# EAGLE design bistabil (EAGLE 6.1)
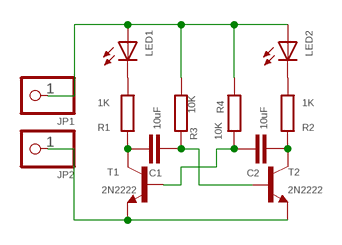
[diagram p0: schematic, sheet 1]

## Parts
C1  10uF  C-EU025-030X050  [C025-030X050]
C2  10uF  C-EU025-030X050  [C025-030X050]
JP1  PINHD-1X1  [1X01]
JP2  PINHD-1X1  [1X01]
LED1  LED3MM  [LED3MM]
LED2  LED3MM  [LED3MM]
R1  1K  R-EU_0204/7  [0204/7]
R2  1K  R-EU_0204/7  [0204/7]
R3  10K  R-EU_0204/7  [0204/7]
R4  10K  R-EU_0204/7  [0204/7]
T1  2N2222  [TO92-EBC-OVAL]
T2  2N2222  [TO92-EBC-OVAL]

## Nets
GND: JP2.1 T1.E T2.E
N$1: C1.1 R1.1 T1.C
N$2: LED1.K(C) R1.2
N$3: C2.2 R2.1 T2.C
N$5: C2.1 R4.1 T1.B
N$6: LED2.K(C) R2.2
N$8: JP1.1 LED1.A LED2.A R3.2 R4.2
N$12: C1.2 R3.1 T2.B

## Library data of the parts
C1 C2 = rcl:C-EU: CAPACITOR, European symbol
JP1 JP2 = pinhead:PINHD-1X1: PIN HEADER
LED1 LED2 = adafruit:LED: LED
R1-R4 = resistor:R-EU_: RESISTOR, European symbol
T1 T2 = adafruit:2N2222: NPN TRANSISTOR Big oval pads

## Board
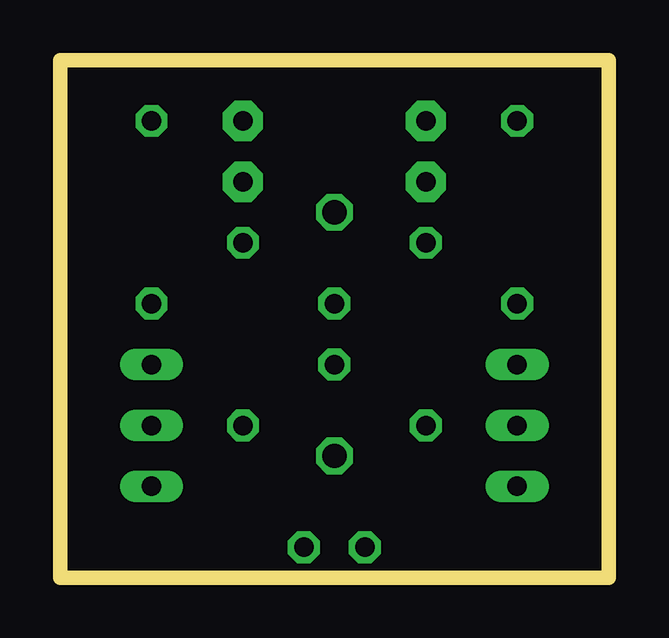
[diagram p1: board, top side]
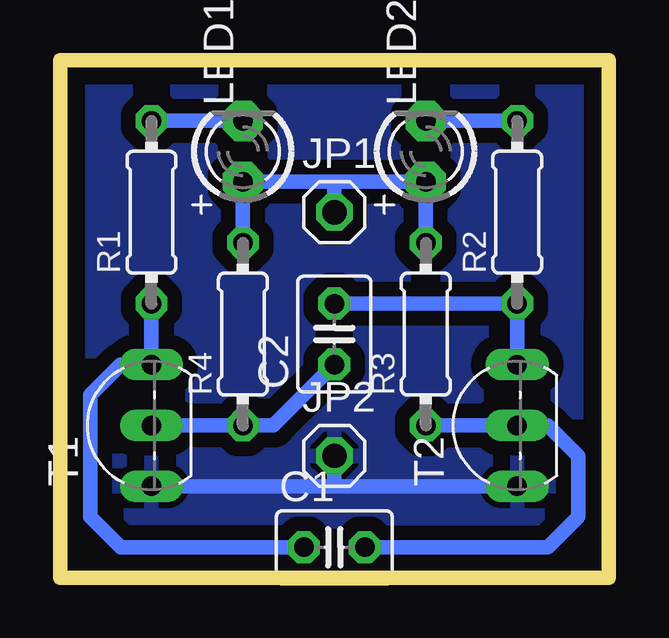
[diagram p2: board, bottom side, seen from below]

Size 22.86 x 21.59 mm. Coordinates in mm from the lower left corner, seen from the top.
Outline: 22.86,0 0.02,0 0,21.59 22.86,21.59 22.86,0
Copper layers (1*16): Top 0.035mm / dielectric 1.5mm / Bottom 0.035mm
Design rules: minimum track width 10mil, minimum drill 24mil, track to track 8mil, track to pad 8mil, pad to pad 8mil, via to via 8mil, smd to smd 8mil, copper to edge 40mil, drill to drill 8mil, minimum pad ring 10mil, minimum via ring 8mil, stop-mask expansion 4mil, vias tented up to drill 0mil, thermal gap 10mil
Milling: 4 lines

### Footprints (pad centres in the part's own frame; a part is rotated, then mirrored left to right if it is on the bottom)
C025-030X050 = drill 0.813 octagon: 1 -1.27,0; 2 1.27,0
1X01 = drill 1.016 octagon: 1 0,0
LED3MM = drill 0.813 pad 1.676 octagon: A -1.27,0; K 1.27,0
0204/7 = drill 0.813 octagon: 1 -3.81,0; 2 3.81,0
TO92-EBC-OVAL = drill 0.813 long: B 0,-1.27; C 2.54,-1.27; E -2.54,-1.27

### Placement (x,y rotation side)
C1  11.43,1.27 0 bottom
C2  11.43,10.16 90 bottom
JP1  11.43,15.24 0 bottom
JP2  11.43,5.08 0 bottom
LED1  15.24,17.78 90 bottom
LED2  7.62,17.78 90 bottom
R1  19.05,15.24 90 bottom
R2  3.81,15.24 90 bottom
R3  7.62,10.16 90 bottom
R4  15.24,10.16 90 bottom
T1  20.32,6.35 90 bottom
T2  5.08,6.35 90 bottom

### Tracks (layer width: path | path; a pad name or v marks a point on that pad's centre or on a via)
GND
  Bottom 0.61: T1.E 11.43,3.81 | 11.43,3.81 T2.E | JP2.1 11.43,3.81
  pour Bottom (isolate 0.61): 22.86,21.59 22.86,0 0,0 0,21.59
N$1
  Bottom 0.61: R1.1 T1.C 20.32,8.89 21.59,7.62 21.59,2.54 20.32,1.27 C1.1
N$2
  Bottom 0.61: R1.2 LED1.K
N$3
  Bottom 0.61: C2.2 R2.1 T2.C
N$5
  Bottom 0.61: T1.B R4.1 13.97,6.35 C2.1
N$6
  Bottom 0.61: LED2.K R2.2
N$8
  Bottom 0.61: R4.2 LED1.A 11.43,16.51 | R3.2 LED2.A 11.43,16.51 | JP1.1 11.43,16.51
N$12
  Bottom 0.61: R3.1 T2.B 2.54,6.35 1.27,5.08 1.27,2.54 2.54,1.27 C1.2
